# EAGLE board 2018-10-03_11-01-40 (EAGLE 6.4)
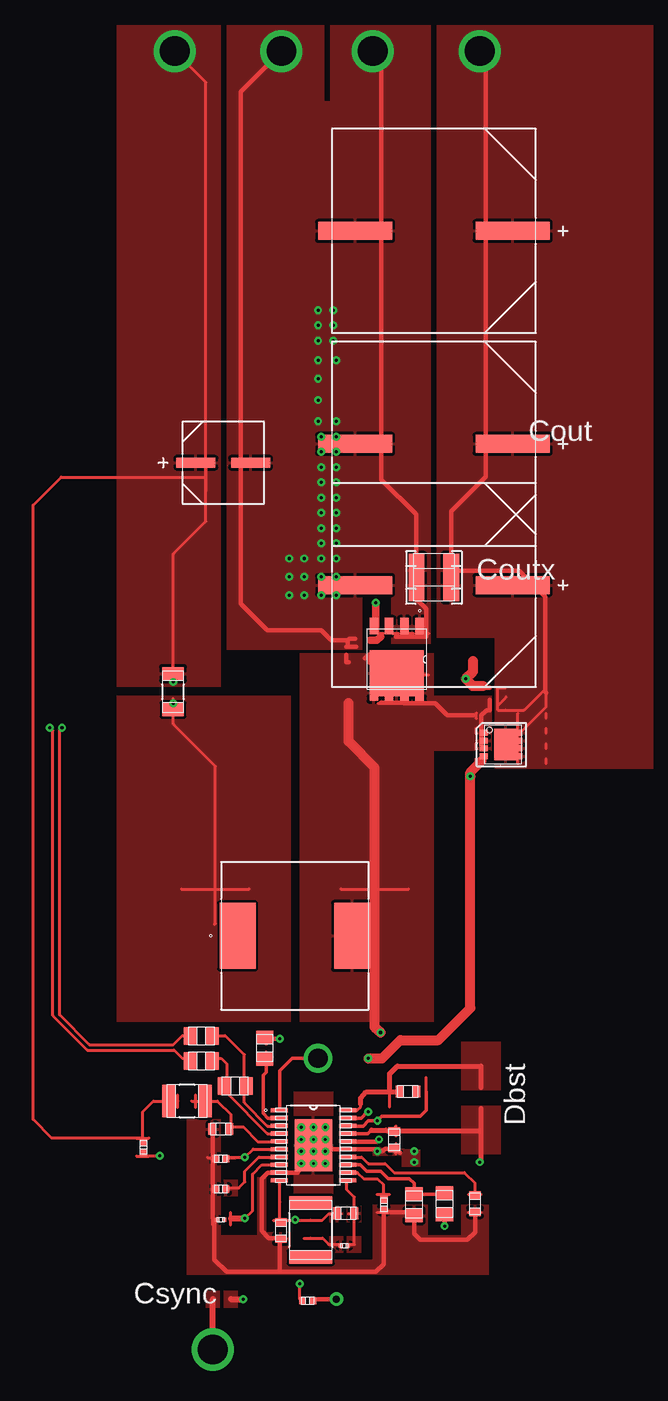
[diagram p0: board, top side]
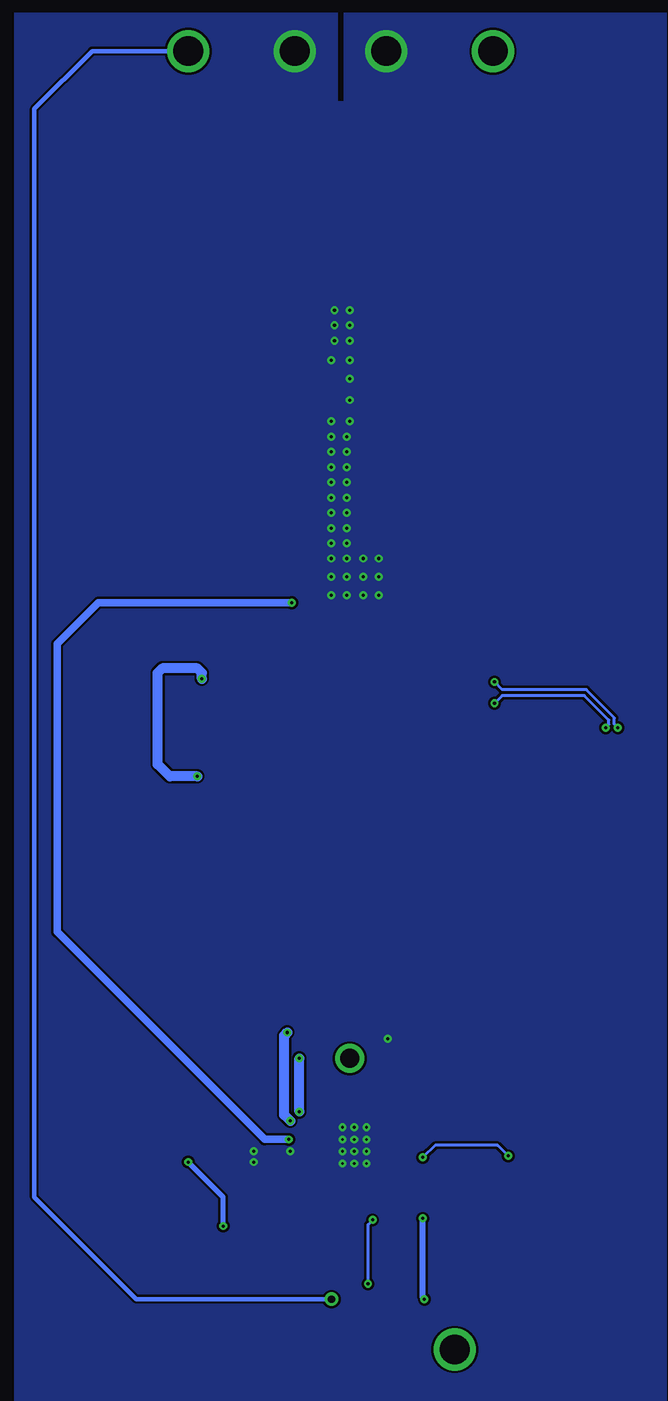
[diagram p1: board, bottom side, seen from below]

No outline drawn. Coordinates in mm, seen from the top.
Copper layers ((1*2)+(15*16)): TOP / INTERNAL1 / layer 15 / BOTTOM

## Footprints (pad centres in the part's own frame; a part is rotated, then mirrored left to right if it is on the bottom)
0603 = smd 0.66 x 0.965: 1 -0.699,0; 2 0.699,0
1812 = smd 1.067 x 3.607: 1 -2.273,0; 2 2.273,0
0805 = smd 1.118 x 1.448: 1 -0.902,0; 2 0.902,0
CAPSMT_62_C10 = smd 3.251 x 0.813: 1 -2.273,0; 2 2.273,0
SM_RADIAL_J16 = smd 6.172 x 1.499: 1 -6.566,0; 2 6.566,0
1210_270 = smd 1.3 x 2.7: 1 -1.45,0; 2 1.45,0
0402 = smd 0.559 x 0.61: 1 -0.419,0; 2 0.419,0
TP-1502 = drill 0.813 round: 1 0,0
MSS1210 = smd 2.997 x 5.512: 1 -4.763,0; 2 4.763,0
TRANS_NexFET_Q5B = smd 1.37 x 0.71: 1 -2.77,1.905; 2 -2.77,0.635; 3 -2.77,-0.635; 4 -2.77,-1.905; 5 2.77,-1.905; 6 2.77,-0.635; 7 2.77,0.635; 8 2.77,1.905 | smd 3.85 x 4.52: 9 1.16,0
DNH0008A = smd 0.68 x 0.5: 1 -1.625,0.975; 2 -1.625,0.325; 3 -1.625,-0.325; 4 -1.625,-0.975 | smd 0.41 x 0.5: 5 1.385,-0.975; 6 1.385,-0.325; 7 1.385,0.325; 8 1.385,0.975 | smd 1.96 x 2.65: 9 0.205,0
0201 = smd 0.356 x 0.33: 1 -0.292,0; 2 0.292,0
1206 = smd 1.118 x 1.803: 1 -1.499,0; 2 1.499,0
1210 = smd 1.118 x 2.692: 1 -1.499,0; 2 1.499,0
MXA20A = smd 1.422 x 0.356: 1 -2.845,2.925; 2 -2.845,2.275; 3 -2.845,1.625; 4 -2.845,0.975; 5 -2.845,0.325; 6 -2.845,-0.325; 7 -2.845,-0.975; 8 -2.845,-1.625; 9 -2.845,-2.275; 10 -2.845,-2.925; 11 2.845,-2.925; 12 2.845,-2.275; 13 2.845,-1.625; 14 2.845,-0.975; 15 2.845,-0.325; 16 2.845,0.325; 17 2.845,0.975; 18 2.845,1.625; 19 2.845,2.275; 20 2.845,2.925 | smd 3.15 x 4.343: 21 0,0

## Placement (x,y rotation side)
Cbst  [0603]  60.07,56.67 0 top
Ccomp  [1812]  51.97,45.14 270 top
Ccomp2  [0603]  54.89,46.53 0 top
Ccs  [0805]  45.67,57.15 180 top
Cin  [CAPSMT_62_C10]  44.68,109.07 0 top
Cout_1  [SM_RADIAL_J16]  62.23,110.64 180 top
Cout_2  [SM_RADIAL_J16]  62.23,128.4 180 top
Cout_3  [SM_RADIAL_J16]  62.23,98.88 180 top
Cout_4  [SM_RADIAL_J16]  62.23,98.88 180 top
Coutx_1  [1210_270]  62.23,98.88 180 top
Coutx_2  [1210_270]  62.23,98.88 180 top
Coutx_3  [1210_270]  62.23,98.88 180 top
Coutx_4  [1210_270]  62.23,100.13 180 top
Cres  [0603]  65.66,47.32 270 top
Css  [0402]  44.48,48.54 180 top
Cvcc  [0603]  58.93,52.65 90 top
Cvin  [0603]  44.48,53.54 180 top
GND  [TP-1502]  49.48,143.36 180 top
GND1  [TP-1502]  57.15,143.36 180 top
L1  [MSS1210]  50.65,69.65 0 top
M1  [TRANS_NexFET_Q5B]  59.13,92.68 270 top
M2  [DNH0008A]  68.02,85.6 0 top
Rcomp  [0201]  54.76,43.84 180 top
Rcsfn  [0805]  42.85,61.29 180 top
Rcsfp  [0805]  42.85,59.23 180 top
Rfbb  [0603]  49.48,45.09 270 top
Rfbt  [0402]  51.71,39.24 180 top
Rmodeb  [0805]  60.58,47.24 270 top
Rmodet  [0805]  63.12,47.32 270 top
Ropt  [0805]  48.13,60.3 90 top
Rs  [1206]  40.49,89.99 270 top
Rslope  [0402]  58.06,47.24 270 top
Rt  [0201]  44.48,45.97 180 top
Ruvb  [0402]  44.48,51.08 180 top
Ruvt  [0402]  38.02,52.02 270 top
Rvin  [1210]  41.66,55.88 0 top
SYNCOUT  [TP-1502]  52.58,59.59 0 top
U1  [MXA20A]  52.2,52.2 0 top
VIN  [TP-1502]  40.61,143.36 180 top
VOUT  [TP-1502]  66.01,143.36 180 top
Vsync  [TP-1502]  43.71,35.23 0 top

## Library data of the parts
Cbst = ultra-librarian; RefDes: Cbst; Type: C1608X5R1H334K080AB
Ccomp = ultra-librarian; RefDes: Ccomp; Type: C1812C273J5GACTU
Ccomp2 = ultra-librarian; RefDes: Ccomp2; Type: GCM1885C1H152JA16D
Ccs = ultra-librarian; RefDes: Ccs; Type: 08051A100CAT2A
Cin = ultra-librarian; RefDes: Cin; Type: 16SVPG270M
Cout_1-Cout_4 Coutx_1-Coutx_4 = ultra-librarian
Cres = ultra-librarian; RefDes: Cres; Type: GRM188R71E474KA12D
Css = ultra-librarian; RefDes: Css; Type: GRM155R61A224KE19D
Cvcc = ultra-librarian; RefDes: Cvcc; Type: C1608X6S1C475K080AC
Cvin = ultra-librarian; RefDes: Cvin; Type: GRM188R61C474KA93D
GND = ultra-librarian; RefDes: GND; Type: TP-1502
GND1 = ultra-librarian; RefDes: GND1; Type: TP-1502
L1 = ultra-librarian; RefDes: L1; Type: MSS1210-683MEB
M1 = ultra-librarian; RefDes: M1; Type: CSD18532Q5B
M2 = ultra-librarian; RefDes: M2; Type: CSD18543Q3A
Rcomp = ultra-librarian; RefDes: Rcomp; Type: RC0201FR-0736K5L
Rcsfn = ultra-librarian; RefDes: Rcsfn; Type: 08051A100CAT2A
Rcsfp = ultra-librarian; RefDes: Rcsfp; Type: 08051A100CAT2A
Rfbb = ultra-librarian; RefDes: Rfbb; Type: RC0603FR-071K6L
Rfbt = ultra-librarian; RefDes: Rfbt; Type: CRCW040246K4FKED
Rmodeb = ultra-librarian; RefDes: Rmodeb; Type: 08051A100CAT2A
Rmodet = ultra-librarian; RefDes: Rmodet; Type: 08051A100CAT2A
Ropt = ultra-librarian; RefDes: Ropt; Type: 08051A100CAT2A
Rs = ultra-librarian; RefDes: Rs; Type: 12061A100JAT2A
Rslope = ultra-librarian; RefDes: Rslope; Type: CRCW0402301KFKED
Rt = ultra-librarian; RefDes: Rt; Type: RC0201FR-07162KL
Ruvb = ultra-librarian; RefDes: Ruvb; Type: CRCW04028K25FKED
Ruvt = ultra-librarian; RefDes: Ruvt; Type: CRCW040251K1FKED
Rvin = ultra-librarian; RefDes: Rvin; Type: RC1210FR-072R74L
SYNCOUT = ultra-librarian; RefDes: SYNCOUT; Type: TP-1502
U1 = ultra-librarian; RefDes: U1; Type: LM5122MH/NOPB
VIN = ultra-librarian; RefDes: VIN; Type: TP-1502
VOUT = ultra-librarian; RefDes: VOUT; Type: TP-1502
Vsync = ultra-librarian; RefDes: Vsync; Type: TP-1502

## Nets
0: Cin.2 Cout_1.2 Cout_2.2 Cout_3.2 Cout_4.2 Coutx_1.2 Coutx_2.2 Coutx_3.2 Coutx_4.2 Cres.2 Css.2 Cvcc.1 Cvin.2 GND1.1 GND.1 M1.1 M1.2 M1.3 Rfbb.2 Rmodeb.1 Rmodeb.2 Rmodet.1 Ropt.1 Ropt.2 Rslope.2 Rt.2 Ruvb.2 U1.2 U1.9 U1.13 U1.15 U1.21
1: Ruvb.1 Ruvt.2 U1.6
2: Cvin.1 Rvin.2 U1.5
3: Rslope.1 U1.12
4: Ccs.2 Cin.1 Rcsfp.1 Rcsfp.2 Rs.1 Ruvt.1 Rvin.1 U1.4 VIN.1
5: Ccs.1 L1.1 Rcsfn.1 Rcsfn.2 Rs.2 U1.3
6: Rt.1 U1.8
7: Cvcc.2 Rmodet.2 U1.17
8: Cbst.1 U1.20
9: Css.1 U1.7
10: Cres.1 U1.14
11: Ccomp2.1 Ccomp.1 Rfbb.1 Rfbt.2 U1.10
12: M2.4 U1.19
13: M1.4 U1.16
14: Ccomp2.2 Rcomp.1 U1.11
15: Cout_1.1 Cout_2.1 Cout_3.1 Cout_4.1 Coutx_1.1 Coutx_2.1 Coutx_3.1 Coutx_4.1 M2.5 M2.6 M2.7 M2.8 M2.9 Rfbt.1 VOUT.1
16: Cbst.2 L1.2 M1.5 M1.6 M1.7 M1.8 M1.9 M2.1 M2.2 M2.3 U1.18 Vsync.1
37: Ccomp.2 Rcomp.2
58: SYNCOUT.1 U1.1

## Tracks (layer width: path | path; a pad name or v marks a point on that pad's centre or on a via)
0  (via drill 0.23 pad 0.58, 0.25 pad 0.61, 2.49 pad 3.48)
  TOP 0.254: 51.18,50.19 v51.18,50.67 | 59.07,51.49 59.07,52.32 | 57.51,46.6 58.55,46.6 | 48.87,44.44 49.91,44.44 | 46.14,106.7 46.14,109.04 | 57.87,110.54 57.87,112.17 | 50.85,52.18 53.49,52.18 | 43.38,51.17 44.22,51.17 | 43.8,45.57 43.8,46.61 | 65.13,46.6 66.17,46.6 | 47.73,61.05 48.77,61.05 | 47.73,59.55 48.77,59.55 | 61.34,94.86 61.82,94.86 | 60.07,94.86 60.55,94.86 | 58.8,94.86 59.28,94.86
  TOP 0.305: 49.38,54.46 48.39,54.46 48.01,54.86 48.01,58.04 48.26,58.29 48.26,59.56 48.26,59.94 | 50.9,49.91 51.18,50.19 | 54.99,50.57 56.08,50.57 56.64,50.04 57.78,50.04 58.42,49.4 60.2,49.4 60.58,49.02 60.58,48.11 63.12,48.11
  TOP 0.356: 49.53,41.66 57.4,41.66 58.04,42.29 58.04,46.61 60.58,46.61 60.58,44.83 61.09,44.32 65.02,44.32 65.66,44.96 Cres.2 | 49.53,41.66 44.96,41.66 43.94,42.67 43.94,45.97 43.81,46.1 | 49.53,41.66 49.4,41.78 49.4,44.45 48.49,44.45 47.88,45.09 47.88,49.4 48.39,49.91 49.38,49.91 50.9,49.91 | 43.81,46.1 | 43.81,46.1 43.81,48.64 | 43.81,48.64 | 43.81,48.64 43.81,51.18 | 43.81,51.18 | 43.81,51.18 43.81,53.72 | v57.15,143.38 57.86,142.65 57.86,111.38 57.86,107.67 60.76,104.78 60.76,100.08 60.76,97.71 61.59,96.9 61.59,94.56 60.33,94.56 59.05,94.56 | v49.53,143.38 46.15,140 46.15,107.87 46.15,97.33 48.36,95.12 52.83,95.12 53.67,94.28 55.04,94.28 | v53.19,51.69 53.37,51.87 54.99,51.87 57.35,51.87 v57.53,51.69 57.91,51.69 58.17,51.92 59.05,51.92 | 59.36,51.56 59.44,51.56 | 48.26,61.06 v49.4,61.06 | v49.4,61.06 | 48.26,61.06 | 48.26,60.71 48.26,61.06 | 55.04,94.28 55.04,93.83 54.94,93.73 | 55.04,93.73 55.78,93.73 | 55.68,94.41 55.17,94.41 55.04,94.28
  other vias: 50.16,98.04 51.44,98.04 53.85,121.79 52.58,119.25 50.16,99.57 51.44,99.57 52.58,116.08 52.58,114.3 52.58,112.52 52.58,117.6 54.1,111.25 54.1,109.98 54.1,108.71 54.1,104.9 52.83,104.9 54.1,106.17 54.1,98.04 54.1,101.09 60.58,51.69 60.58,50.8 52.83,109.98 52.83,107.44 52.83,106.17 52.83,108.71 54.1,103.63 54.1,102.36 54.1,99.57 54.1,107.44 54.1,112.52 54.1,117.6 50.16,101.09 52.83,103.63 52.83,99.57 51.44,101.09 52.83,102.36 52.83,98.04 52.58,120.52 52.58,121.79 52.83,101.09 53.85,120.52 53.85,119.25 52.83,111.25 52.2,52.68 53.19,52.68 52.2,51.69 52.2,50.67 53.19,50.67 51.18,51.69 51.18,52.68 51.18,53.7 53.19,53.7 52.2,53.7
  pour TOP (rank 5): 48.87,54.28 48.87,54.61 49.76,54.61 49.76,54.28
  pour TOP (rank 6): 48.87,49.73 48.87,50.06 49.76,50.06 49.76,49.73
  pour TOP (rank 6): 54.46,51.69 54.46,52.02 55.35,52.02 55.35,51.69
  pour TOP (rank 6): 54.46,50.39 54.46,50.72 55.35,50.72 55.35,50.39
  pour TOP (rank 6): 50.55,56.64 53.85,56.64 53.85,47.75 50.55,47.75
  pour TOP (rank 6): 61.09,51.82 61.09,50.42 59.56,50.42 59.56,51.31 57.15,51.31 57.15,52.07
  pour TOP: 44.96,93.47 56.26,93.47 56.26,98.17 58.67,98.17 58.67,93.98 61.98,93.98 61.98,145.54 53.59,145.54 53.59,139.19 53.09,139.19 53.09,145.54 44.96,145.54
  pour TOP: 66.8,41.4 41.66,41.4 41.66,54.36 44.45,54.36 44.45,44.7 47.5,44.7 47.5,49.53 48.26,49.53 48.26,44.96 50.29,44.96 50.29,42.67 57.15,42.67 57.15,47.24 61.72,47.24 61.72,44.7 64.52,44.7 64.52,47.24 66.8,47.24
  pour BOTTOM (rank 6): 26.16,146.56 53.09,146.56 53.09,139.19 53.59,139.19 53.59,146.56 80.52,146.56 80.52,26.16 26.16,26.16
1  (via drill 0.25 pad 0.61)
  TOP 0.254: 44.83,51.18 | 44.83,51.18 45.31,51.18 v46.48,51.18 | v46.48,51.18 | v46.48,51.18 47.17,51.87 49.38,51.87 | v39.37,51.31 39.34,51.31 37.97,51.31 37.97,51.69 | 37.97,51.69 | 37.44,51.3 38.48,51.3 | 44.88,51.17 45.72,51.17
  BOTTOM 0.254: v46.48,51.18 45.47,52.2 40.26,52.2 v39.37,51.31
  pour TOP (rank 2): 48.87,51.69 48.87,52.02 49.76,52.02 49.76,51.69
2
  TOP 0.254: 49.38,52.5 47.55,52.5 46.35,53.72 45.31,53.72 | 45.31,53.72 45.34,53.72 45.34,54.74 44.2,55.88 42.39,55.88 42.04,55.88 | 44.96,53.72 45.31,53.72 | 44.96,53.72 | 42.04,55.88 | 42.38,55.35 42.38,56.39
  pour TOP: 48.87,52.32 48.87,52.65 49.76,52.65 49.76,52.32
3
  TOP 0.254: 58.04,48.11 58.04,48.9 57.53,49.4 56.39,49.4 55.85,49.91 54.99,49.91 | 58.04,47.62 | 58.04,47.62 58.04,48.11 | 58.04,48.11 | 57.51,48.09 58.55,48.09
  pour TOP (rank 3): 54.46,49.73 54.46,50.06 55.35,50.06 55.35,49.73
4  (via drill 0.25 pad 0.61, 0.25 pad 0.66, 2.49 pad 3.48)
  TOP 0.254: 43.23,107.87 43.23,104.19 40.51,101.47 40.51,91.44 | v40.64,143.38 43.23,140.77 43.23,107.87 | 43.23,107.87 31.17,107.87 28.83,105.54 28.83,54.36 30.35,52.81 37.97,52.81 37.97,54.99 38.86,55.88 40.89,55.88 | 49.38,53.16 48.36,53.16 45.01,56.52 45.01,58.93 44.5,59.44 43.66,59.44 | 42.16,59.44 41.27,59.44 40.59,60.12 33.35,60.12 30.48,62.99 30.48,86.74 v30.23,87 | 40.89,55.88 | 43.24,106.7 43.24,109.04 | 40.5,90.6 40.5,92.23 | 40.88,55.35 40.88,56.39 | 37.44,52.79 38.48,52.79 | 44.95,56.87 44.95,57.91 | 42.15,58.9 42.15,59.94 | 43.65,58.9 43.65,59.94
  BOTTOM 0.254: v30.23,87 30.53,87.3 30.53,87.81 32.87,90.17 39.88,90.17 v40.51,90.81
  pour TOP: 48.87,52.98 48.87,53.31 49.76,53.31 49.76,52.98
  pour TOP (rank 5): 44.45,90.42 35.81,90.42 35.81,145.54 44.45,145.54
5
  TOP 0.254: 49.38,53.8 48.36,53.8 46.43,55.75 46.43,59.74 44.83,61.34 43.66,61.34 | 46.44,56.87 46.44,57.91 | 43.65,60.81 43.65,61.85
  pour TOP: 48.87,53.64 48.87,53.98 49.76,53.98 49.76,53.64
6  (via drill 0.25 pad 0.61, 0.25 pad 0.66)
  TOP 0.254: v46.48,46.1 47.12,46.74 47.12,49.78 47.9,50.57 49.38,50.57 | 43.94,70.61 44.02,70.69 44.02,73.56 44.02,83.77 40.51,87.3 40.51,88.62 | 42.34,61.34 41.27,61.34 40.51,60.58 33.53,60.58 31.04,63.07 31.04,86.79 v31.24,87 | 40.5,87.81 40.5,89.43 | 41.2,73.53 46.84,73.53 | 45.3,45.57 45.3,46.61 | 42.15,60.81 42.15,61.85
  TOP 0.508: v46.35,39.37 | 45.31,39.37 v46.35,39.37 | 45.31,46.1 v46.48,46.1
  BOTTOM 0.254: v40.51,89.03 39.88,89.66 33.02,89.66 30.99,87.63 30.99,87.25 v31.24,87
  BOTTOM 0.508: v46.48,46.1 46.48,39.5 v46.35,39.37
  pour TOP: 44.7,38.66 44.7,40.06 45.9,40.06 45.9,38.66
  pour TOP (rank 2): 48.87,50.39 48.87,50.72 49.76,50.72 49.76,50.39
  pour TOP (rank 5): 35.81,89.66 50.29,89.66 50.29,62.48 35.81,62.48
7  (via drill 0.25 pad 0.61)
  TOP 0.254: 59.07,52.98 59.07,53.82
  TOP 0.305: 57.02,53.47 56.72,53.16 54.99,53.16
  TOP 0.356: v63.12,45.47 | v63.12,45.47 63.12,46.61 | 63.12,46.61
  TOP 0.406: 57.02,53.47 58.24,53.47 58.29,53.42 59.05,53.42 66.12,53.42 66.17,53.47 | v66.04,50.8 66.17,50.93 66.17,53.47 | 66.17,53.47 66.17,55.24
  BOTTOM 0.406: v63.12,45.47 63.12,47.88 v66.04,50.8
  pour TOP (rank 3): 54.46,52.98 54.46,53.31 55.35,53.31 55.35,52.98
  pour TOP (rank 5): 64.52,51.44 64.52,55.5 67.79,55.5 67.79,51.44
8
  TOP 0.254: 56.13,55.63 | 56.13,55.63 56.13,55.37 55.85,55.12 54.99,55.12 | 58.55,55.4 58.55,57.84
  TOP 0.406: 59.31,56.77 59.18,56.64 58.55,56.64 | 58.55,56.64 58.55,58.17 59.18,58.8 66.17,58.8 66.17,57.02 | 58.55,56.64 56.62,56.64 56.13,56.13 56.13,55.63
  pour TOP (rank 2): 54.46,54.94 54.46,55.27 55.35,55.27 55.35,54.94
  pour TOP (rank 4): 64.52,56.77 64.52,60.83 67.79,60.83 67.79,56.77
9
  TOP 0.254: 44.83,48.64 | 44.83,48.64 45.31,48.64 45.97,48.64 46.48,49.15 46.48,50.04 47.65,51.21 49.38,51.21
  pour TOP (rank 2): 48.87,51.03 48.87,51.36 49.76,51.36 49.76,51.03
  pour TOP (rank 4): 44.7,47.93 44.7,49.33 45.9,49.33 45.9,47.93
10
  TOP 0.254: 65.66,47.75 | 65.66,47.75 65.66,48.11 65.66,49.02 64.77,49.91 58.93,49.91 58.17,50.67 56.77,50.67 56.21,51.21 54.99,51.21 | 65.13,48.09 66.17,48.09
  pour TOP (rank 3): 54.46,51.03 54.46,51.36 55.35,51.36 55.35,51.03
11  (via drill 0.25 pad 0.61, 0.25 pad 0.66)
  TOP 0.254: 51.44,39.37 | 51.44,39.37 51.05,39.37 51.05,40.62 v51.05,40.64 | 54.48,46.48 | 54.48,46.48 54.1,46.48 53.47,46.48 52.93,45.95 51.94,45.95 50.67,45.95 v50.67,45.97 50.65,45.95 49.4,45.95 49.4,47.47 49.38,47.5 | 49.38,47.5 49.38,49.25 | 49.38,46.33 49.38,47.5 | 48.87,45.94 49.91,45.94 | 51.41,45.94 52.45,45.94
  BOTTOM 0.254: v51.05,40.64 51.05,45.59 v50.67,45.97
  pour TOP (rank 2): 48.87,49.07 48.87,49.4 49.76,49.4 49.76,49.07
  pour TOP (rank 4): 53.49,45.77 53.49,47.17 54.69,47.17 54.69,45.77
12  (via drill 0.25 pad 0.61, 0.25 pad 0.66)
  TOP 0.254: 65.77,83.95 65.77,84.43
  TOP 0.305: 54.99,54.46 56.19,54.46 56.69,54.99
  TOP 0.356: 66.9,90.32 66.5,90.32 66.34,90.47
  TOP 0.813: v56.77,59.44 57.91,59.44 59.44,60.96 62.61,60.96 65.28,63.63 v65.28,82.93 65.28,83.26 66.19,84.2 | 66.34,90.47 65.46,90.47 v64.9,91.06 65.51,91.67 65.51,92.56
  BOTTOM 0.813: v56.77,54.99 v56.77,59.44 | v64.9,91.06 64.9,91.57 65.28,91.95 68.2,91.95 68.58,91.57 68.58,83.95 67.56,82.93 v65.28,82.93
  pour TOP (rank 2): 54.46,54.28 54.46,54.61 55.35,54.61 55.35,54.28
13  (via drill 0.25 pad 0.61, 0.25 pad 0.66)
  TOP 0.254: 57.53,94.86 58.01,94.86
  TOP 0.356: v57.66,52.68 57.48,52.5 54.99,52.5
  TOP 0.61: 57.38,95.12 57.38,97.38 v57.4,97.41 | 56.95,94.28 57.48,94.28 57.78,94.56
  BOTTOM 0.61: v57.4,97.41 73.53,97.41 76.96,93.98 76.96,69.98 59.66,52.68 v57.66,52.68
  pour TOP (rank 3): 54.46,52.32 54.46,52.65 55.35,52.65 55.35,52.32
14
  TOP 0.254: 55.12,43.94 | 55.12,43.94 55.6,43.94 55.6,46.48 | 55.12,46.48 | 55.12,46.48 55.6,46.48 | 54.99,49.25 54.99,48.49 55.6,47.88 55.6,46.48
  pour TOP (rank 3): 54.46,49.07 54.46,49.4 55.35,49.4 55.35,49.07
  pour TOP (rank 4): 54.99,45.77 54.99,47.17 56.18,47.17 56.18,45.77
  pour TOP (rank 4): 54.99,43.23 54.99,44.63 56.18,44.63 56.18,43.23
15  (via drill 0.61 pad 1.12, 2.49 pad 3.48)
  TOP 0.254: 71.5,90.19 69.75,88.47 68.2,88.47 67.56,88.47 67.56,88.82 | 71.58,89.92 71.58,88.72 68.96,86.11 69.24,86.11 | 68.2,90.32 67.56,90.32 67.56,88.82 | 67.56,88.82 68.25,89.53 | 66.56,110.54 66.56,112.17 | 69.23,84 69.23,88.19 | 71.59,87.81 71.59,88.19 | 71.59,86.54 71.59,86.92 | 71.59,85.27 71.59,85.65 | 71.59,84 71.59,84.38 | v54.1,39.37
  TOP 0.356: v66.04,143.38 66.57,142.82 66.57,111.38 66.57,107.92 63.68,105.03 63.68,100.08 69.34,100.08 71.5,97.92 71.5,90.19 71.5,89.99 71.58,89.92 | 52.55,39.37 v54.1,39.37
  BOTTOM 0.356: v66.04,143.38 74.04,143.38 78.87,138.56 78.87,47.88 70.36,39.37 v54.1,39.37 | v54.1,39.37
  pour TOP (rank 5): 62.48,145.54 62.48,94.49 67.31,94.49 67.31,83.57 80.52,83.57 80.52,145.54
16  (via drill 0.25 pad 0.61, 2.49 pad 3.48)
  TOP 0.254: 61.59,55.4 61.59,57.84 | 54.48,73.53 60.12,73.53 | 57.58,91.4 61.77,91.4 | 61.39,89.01 61.77,89.01 | 60.12,89.01 60.5,89.01 | 58.85,89.01 59.23,89.01 | 57.58,89.01 57.96,89.01 | 65.77,87.76 65.77,88.24 | 65.77,86.49 65.77,86.97 | 65.77,85.22 65.77,85.7
  TOP 0.305: 61.59,56.64 61.59,55.12 61.09,54.61 57.89,54.61 v57.53,54.23 56.77,54.23 56.34,53.8 54.99,53.8
  TOP 0.356: 57.78,89.05 59.69,89.05 | 65.51,88.01 63.35,88.01 62.36,89.03 59.72,89.03 59.69,89.05 | 54.94,93.09 54.94,92.43 55.12,92.43 | 56.46,92.76 56.79,93.09 56.79,92.43 58.67,92.43 59.69,91.44 59.69,89.05 | 66.19,85.47 66.19,86.74 66.19,88.01 66.65,88.47 66.9,88.47 66.9,89.31
  TOP 0.508: v43.81,35.18 | v43.81,35.18 43.81,39.37
  TOP 0.813: v57.78,61.59 57.3,62.05 57.3,73.56 57.3,83.64 55.12,85.85 55.12,89.05
  BOTTOM 0.813: v57.78,61.59 58.04,61.34 58.04,54.74 v57.53,54.23
  pour TOP: 43.21,38.66 43.21,40.06 44.4,40.06 44.4,38.66
  pour TOP (rank 3): 54.46,53.64 54.46,53.98 55.35,53.98 55.35,53.64
  pour TOP (rank 5): 51.05,93.22 62.23,93.22 62.23,89.66 67.06,89.66 67.06,85.09 62.23,85.09 62.23,62.48 51.05,62.48
37
  TOP 0.254: 54.48,43.94 | 54.48,43.94 54.1,43.94 53.47,43.94 52.96,44.45 51.94,44.45 | 51.94,44.45 | 51.41,44.44 52.45,44.44
  pour TOP (rank 4): 53.49,43.23 53.49,44.63 54.69,44.63 54.69,43.23
58  (via drill 1.6 pad 2.21)
  TOP 0.305: 49.38,55.12 49.38,58.4 50.42,59.44 v52.58,59.44
  pour TOP: 48.87,54.94 48.87,55.27 49.76,55.27 49.76,54.94

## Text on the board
ASSYNOTES: Cout | Coutx | Dbst | Csync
